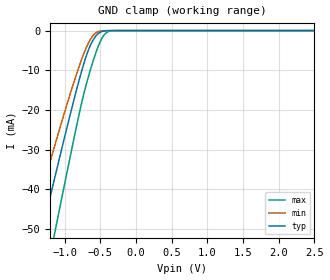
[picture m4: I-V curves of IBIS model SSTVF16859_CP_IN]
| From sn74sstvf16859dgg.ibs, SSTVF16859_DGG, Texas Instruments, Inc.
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[Model]   SSTVF16859_CP_IN
Model_type  Input
Vinh=0.97
Vinl=1.53
| variable   typ   min   max
|C_comp   1.88pF   1.50pF   2.29pF
C_comp   3.12pF   3.07pF   3.17pF
|Note: The above cap values are based on Back-Annotation by Roman Pacheco
[Temperature Range]   40   85   0
| Ambient temperature   25   70   0
[Voltage range]   2.5   2.5   2.5
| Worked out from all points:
|   GND clamp passes 1 mA (typ) near -0.54 V on its own axis
[GND Clamp]
| SSTVF16859_CP_IN
|   Voltage   I(typ)   I(min)   I(max)
-2.5V     -142.5mA   -119mA     -171.5mA
-1.49V    -63.97mA   -51.46mA   -82.34mA
-1.44V    -60.12mA   -48.21mA   -77.9mA
-1.305V   -49.78mA   -39.54mA   -65.87mA
-1.14V    -37.28mA   -29.15mA   -51.17mA
-910mV    -20.37mA   -15.32mA   -30.82mA
-745mV    -9.239mA   -6.51mA    -17.05mA
-650mV    -4.192mA   -2.605mA   -10.64mA
-550mV    -1.134mA   -458.4uA   -5.008mA
-445mV    -115.2uA   -35.68uA   -1.098mA
-325mV    -3.541uA   -1.298uA   -45.32uA
2.5V      338.1pA    223.4pA    3.669nA
